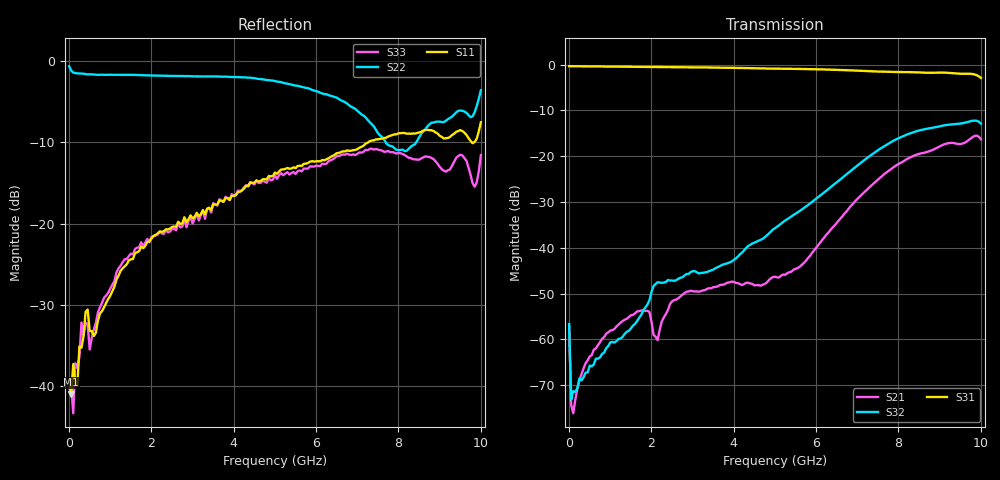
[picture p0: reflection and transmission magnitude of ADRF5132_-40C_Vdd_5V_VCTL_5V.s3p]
! Device:  ADRF5132
! Description: Silicon SPDT Switch
! Frequency:  0.7 -  5 GHz
! Ports:
!	RFC	= Port 1
!	RF1	= Port 2
!  RF2  = Port 3
! Vdd:  5 Volt
! Control:  0/5 Volt
! Data:  Data was collected using a calibrated 4 port network analyzer and de-embedded using AtaiTec's In Situ De-Embedding.
! Note:  Analog Devices supplies this data as a sample of measured data
!  for this product.  Your particular data for this product may vary.
!  Data was taken at -40 degrees C.
!  Analog Devices reserves the right to change this data at anytime.
# GHZ S DB R 50.0
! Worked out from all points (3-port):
!   201 points, 10 MHz to 10 GHz, reference 50 ohm
!   strongest paths, dB at 10 MHz, 2.507 GHz, 5.005 GHz, 7.503 GHz, 10 GHz:
!     S31: -0.3, -0.6, -0.9, -1.5, -2.9
!     S32: -56.7, -47.2, -35.7, -18.7, -12.9
!     S21: -56.9, -51.7, -46.3, -25.1, -16.3
!   lowest |S11| = -41.0 dB at 59.95 MHz (marker M1), VSWR 1.02, Z = 50.9 - j0.164 ohm
!   |S11| at or under -10 dB: start of sweep to 7.264 GHz; 9.782589 GHz to 9.830849 GHz (48.26 MHz wide, 0.492 % of centre)
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0.01  -39.19 -33.6  -56.74 -58.6  -0.34 -0.1
      -56.93 -55.7  -0.63 -8.3  -57.63 -61.9
      -0.34 -0.2  -56.66 -58.6  -40.27 34.9
0.05995  -40.99 -10.4  -75.44 -41.1  -0.35 -1.1
         -74.31 -50.7  -1.17 -42.0  -71.98 -48.9
         -0.36 -1.1  -73.13 -33.9  -39.90 -7.2
0.3097  -35.23 -55.6  -67.48 63.9  -0.34 -5.3
        -67.64 60.5  -1.53 -127.5  -68.56 -35.6
        -0.35 -5.3  -68.94 -38.6  -32.14 -47.0
0.75925  -31.03 -92.4  -60.77 72.6  -0.39 -12.7
         -60.62 72.8  -1.68 -166.3  -63.96 -83.7
         -0.41 -12.7  -63.93 -84.0  -30.25 -78.7
1.75825  -22.80 -133.4  -53.71 56.8  -0.48 -29.0
         -53.68 57.0  -1.73 164.0  -54.68 -116.5
         -0.50 -29.0  -54.67 -116.5  -22.27 -106.5
2.15785  -21.20 -147.7  -59.91 77.2  -0.52 -35.5
         -60.16 75.3  -1.80 156.2  -47.53 -141.7
         -0.54 -35.5  -47.51 -141.7  -21.33 -115.2
2.85715  -19.80 -169.6  -49.63 70.0  -0.57 -46.8
         -49.58 70.1  -1.85 143.3  -45.74 -169.6
         -0.59 -46.8  -45.72 -169.9  -20.43 -117.9
5.005  -13.71 150.4  -46.35 -10.0  -0.87 -82.1
       -46.31 -9.1  -2.47 104.4  -35.68 -177.4
       -0.89 -82.1  -35.72 -177.7  -14.06 -143.5
9.6004  -8.80 61.2  -17.06 62.9  -1.99 -160.0
        -17.09 63.6  -6.21 78.2  -12.71 37.4
        -2.01 -160.1  -12.72 36.9  -11.92 144.8
10  -7.53 22.7  -16.24 13.5  -2.84 179.3
    -16.28 14.3  -3.59 7.6  -12.87 8.4
    -2.89 179.3  -12.89 7.8  -11.56 96.0
